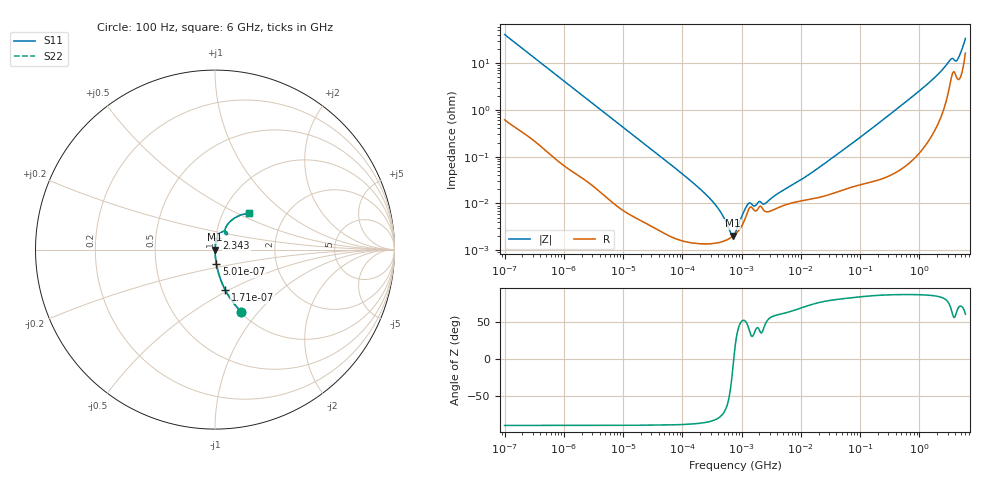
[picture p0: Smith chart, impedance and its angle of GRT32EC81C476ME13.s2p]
!Murata Part Number: GRT32EC81C476ME13
!These Parameters are Measured in Series Mode Connection
!Data Generated on Jun 19, 2026
!  o--ll--o
!Port1  Port2
!  o------o
!Operation Temp=25[degC], DC Bias Voltage=0[V]
!Freq. Start=100[Hz] Stop=6[GHz] 401[Steps]
# Hz S RI R 50
!Freq.(Hz) S11(Real) S11(Imag) S21(Real) S21(Imag) S12(Real) S12(Imag) S22(Real) S22(Imag)
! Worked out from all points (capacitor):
!   401 points, 100 Hz to 6 GHz, reference 50 ohm
!   read as one part in series: C = 38.9 uF near 109 Hz
!   lowest |Z| = 2.04 mohm at 708.2 kHz (marker M1)
!   series resonance near 736 kHz, so ESL is about 1.2 nH
!   S11 on the Smith chart (normalised r, x): 100 Hz: 1.01, -0.81; 171 Hz: 1.01, -0.48; 501 Hz: 1.00, -0.17; 2.343 GHz: 1.01, +0.13; 6 GHz: 1.33, +0.59
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100  0.1461 -0.3457  0.8539 0.3457  0.8539 0.3457  0.1461 -0.3457
171  0.0573 -0.2246  0.9427 0.2246  0.9427 0.2246  0.0573 -0.2246
280  0.0234 -0.1432  0.9766 0.1432  0.9766 0.1432  0.0234 -0.1432
501  0.00809 -0.0819  0.9919 0.0819  0.9919 0.0819  0.00809 -0.0819
2008  0.000789 -0.0209  0.9992 0.0209  0.9992 0.0209  0.000789 -0.0209
40335  2.75e-05 -0.00107  1 0.00107  1 0.00107  2.75e-05 -0.00107
154540  1.43e-05 -0.00027  1 0.00027  1 0.00027  1.43e-05 -0.00027
345986  1.41e-05 -9.94e-05  1 9.94e-05  1 9.94e-05  1.41e-05 -9.94e-05
708247  1.98e-05 -4.8e-06  1 4.8e-06  1 4.8e-06  1.98e-05 -4.8e-06
774597  2.18e-05 6.4e-06  1 -6.4e-06  1 -6.4e-06  2.18e-05 6.4e-06
2481164  6.79e-05 7.19e-05  0.9999 -7.19e-05  0.9999 -7.19e-05  6.79e-05 7.19e-05
4060267  8.03e-05 0.00014  0.9999 -0.00014  0.9999 -0.00014  8.03e-05 0.00014
1.555665e7  0.000125 0.000445  0.9999 -0.000445  0.9999 -0.000445  0.000125 0.000445
8.154455e7  0.000237 0.00211  0.9998 -0.00211  0.9998 -0.00211  0.000237 0.00211
3.124326e8  0.00045 0.00782  0.9996 -0.00782  0.9996 -0.00782  0.00045 0.00782
1.197065e9  0.0025 0.0305  0.9975 -0.0305  0.9975 -0.0305  0.0025 0.0305
2.34314e9  0.0116 0.0659  0.9884 -0.0659  0.9884 -0.0659  0.0116 0.0659
3.352442e9  0.0484 0.1023  0.9516 -0.1023  0.9516 -0.1023  0.0484 0.1023
4.009986e9  0.064 0.083  0.936 -0.083  0.936 -0.083  0.064 0.083
4.385646e9  0.054 0.0972  0.946 -0.0972  0.946 -0.0972  0.054 0.0972
5.016141e9  0.0708 0.1414  0.9292 -0.1414  0.9292 -0.1414  0.0708 0.1414
6e9  0.1916 0.2042  0.8084 -0.2042  0.8084 -0.2042  0.1916 0.2042
